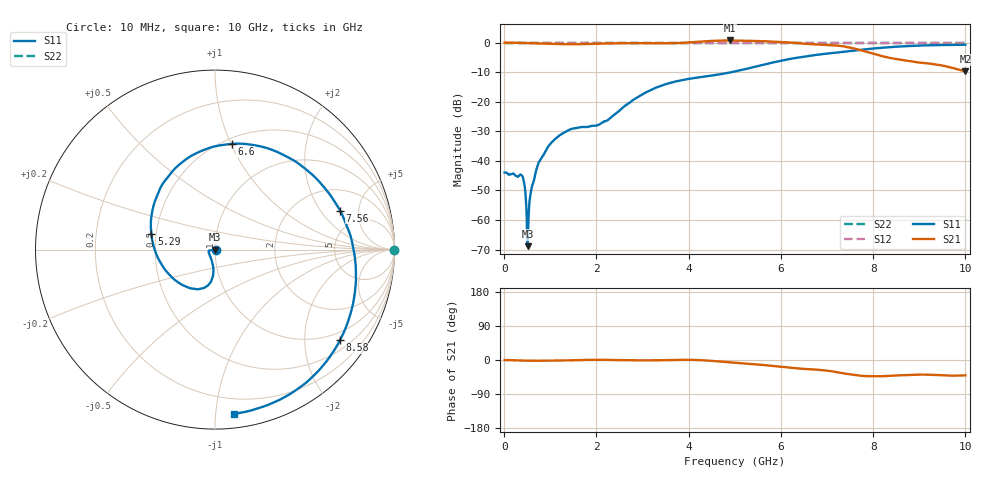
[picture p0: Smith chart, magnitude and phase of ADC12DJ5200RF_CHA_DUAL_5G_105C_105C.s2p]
! Texas Instruments, Inc.
! ADC12DJ5200RF - CH A S-Parameters (Dual Ch Mode, Fs = 5 GSPS, 105 degC case, 105 degC juntion)
! Port 1 represents the 100-ohm differenal input, Port 2 the digital output
! freq  dbS11  angS11  dbS21 angS21 dbS12 angS12 dbS22 angS22
# HZ S DB R 100
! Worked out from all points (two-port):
!   1000 points, 10 MHz to 10 GHz, reference 100 ohm
!   highest |S21| = 0.74 dB at 4.89 GHz (marker M1); lowest = -9.7 dB at 10 GHz (marker M2)
!   |S21| within 3 dB of the highest: start of sweep to 7.66 GHz
!   lowest |S11| = -68.9 dB at 510 MHz (marker M3), VSWR 1.00, Z = 100 - j0.0713 ohm
!   |S11| at or under -10 dB: start of sweep to 4.932 GHz
!   |S22| runs from 0.0 to 0.0 dB; largest |S21 - S12| = 0.78
!   S11 on the Smith chart (normalised r, x): 10 MHz: 1.01, -0.00; 5.29 GHz: 0.47, +0.10; 6.6 GHz: 0.55, +1.01; 7.56 GHz: 3.35, +3.13; 8.58 GHz: 0.75, -2.91; 10 GHz: 0.09, -1.12
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1e7  -43.98 -7.6  0.00 -0.0  0.00 0.0  0.00 0.0
3.8e8  -44.92 -10.5  -0.07 -1.5  0.00 0.0  0.00 0.0
4.3e8  -47.24 -0.5  -0.10 -1.7  0.00 0.0  0.00 0.0
4.7e8  -52.81 6.8  -0.12 -1.8  0.00 0.0  0.00 0.0
5.1e8  -68.87 -81.6  -0.14 -1.9  0.00 0.0  0.00 0.0
7.1e8  -42.37 -157.4  -0.26 -2.0  0.00 0.0  0.00 0.0
9.4e8  -35.52 -169.1  -0.36 -2.0  0.00 0.0  0.00 0.0
1.26e9  -30.80 -171.7  -0.50 -1.4  0.00 0.0  0.00 0.0
1.68e9  -28.56 -163.4  -0.52 -0.0  0.00 0.0  0.00 0.0
2.24e9  -26.25 -119.8  -0.26 0.0  0.00 0.0  0.00 0.0
3.34e9  -14.98 -96.9  -0.24 -0.8  0.00 0.0  0.00 0.0
4.19e9  -11.81 -123.4  0.27 -0.1  0.00 0.0  0.00 0.0
4.89e9  -10.14 -166.0  0.74 -6.2  0.00 0.0  0.00 0.0
5.01e9  -9.74 -174.4  0.70 -7.5  0.00 0.0  0.00 0.0
5.29e9  -8.74 165.9  0.59 -9.9  0.00 0.0  0.00 0.0
5.9e9  -6.49 126.2  0.29 -16.6  0.00 0.0  0.00 0.0
6.6e9  -4.49 81.1  -0.46 -24.1  0.00 0.0  0.00 0.0
6.67e9  -4.33 76.5  -0.54 -24.7  0.00 0.0  0.00 0.0
7.56e9  -2.73 17.4  -1.87 -39.0  0.00 0.0  0.00 0.0
8.34e9  -1.56 -25.8  -5.09 -42.0  0.00 0.0  0.00 0.0
8.58e9  -1.31 -35.9  -5.73 -40.5  0.00 0.0  0.00 0.0
1e10  -0.71 -83.2  -9.71 -40.6  0.00 0.0  0.00 0.0
